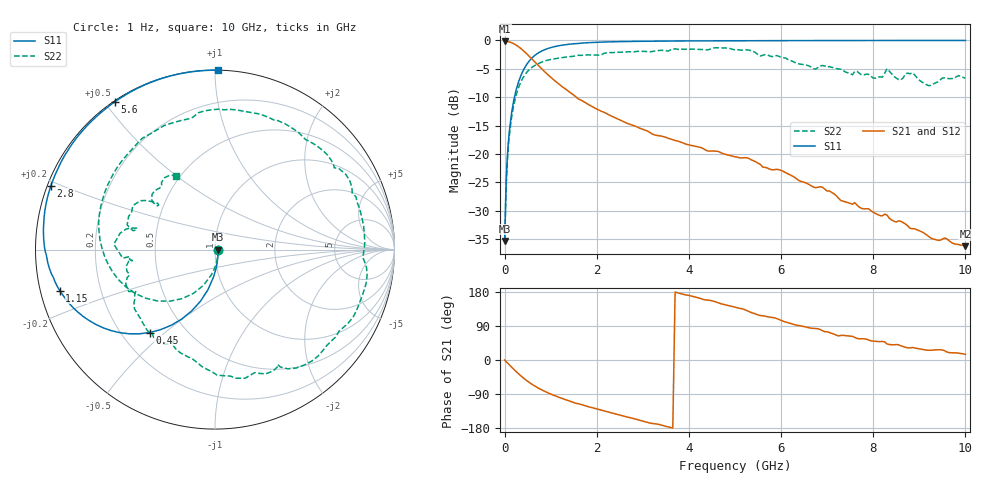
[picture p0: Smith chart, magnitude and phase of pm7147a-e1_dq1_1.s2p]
# GHz S DB R 50
! S-Parameters data
! Freq  dbS11  angS11  dbS21  angS21  dbS12  angS12  dbS22  angS22
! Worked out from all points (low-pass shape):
!   279 points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, 1 Hz to 10 GHz, reference 50 ohm
!   highest |S21| = -0.15 dB at 1.259 kHz (marker M1); lowest = -36.2 dB at 10 GHz (marker M2)
!   |S21| within 3 dB of the highest: start of sweep to 578.2 MHz
!   lowest |S11| = -35.3 dB at 1.585 kHz (marker M3), VSWR 1.03, Z = 51.7 - j0.000223 ohm
!   |S11| at or under -10 dB: start of sweep to 213.7 MHz
!   |S22| runs from -35.3 to -1.3 dB; largest |S21 - S12| = 0
!   S11 on the Smith chart (normalised r, x): 1 Hz: 1.03, -0.00; 450 MHz: 0.31, -0.45; 1.15 GHz: 0.06, -0.13; 2.8 GHz: 0.01, +0.19; 5.6 GHz: 0.00, +0.53; 10 GHz: 0.00, +1.02
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1e-09  -35.30 -0.0  -0.15 -0.0  -0.15 -0.0  -35.30 -0.0
1.2589e-06  -35.30 -0.0  -0.15 -0.0  -0.15 -0.0  -35.30 -0.0
1.5849e-06  -35.30 -0.0  -0.15 -0.0  -0.15 -0.0  -35.30 -0.0
0.03981072  -23.85 -78.0  -0.17 -5.0  -0.17 -5.0  -24.54 -78.8
0.1  -16.21 -93.3  -0.26 -12.5  -0.26 -12.5  -16.95 -98.2
0.25  -8.73 -110.9  -0.81 -30.5  -0.81 -30.5  -9.63 -124.0
0.45  -4.60 -128.3  -2.12 -51.6  -2.12 -51.6  -5.92 -150.9
0.75  -2.11 -148.0  -4.56 -75.4  -4.56 -75.4  -4.00 179.0
1.15  -0.97 -165.2  -7.50 -97.1  -7.50 -97.1  -3.14 149.5
1.7  -0.45 179.5  -10.69 -118.9  -10.69 -118.9  -2.62 117.6
2.8  -0.17 158.7  -14.99 -154.6  -14.99 -154.6  -2.01 65.3
3.35  -0.12 150.6  -16.78 -170.1  -16.78 -170.1  -1.76 42.3
4.2  -0.07 139.5  -18.74 164.2  -18.74 164.2  -1.56 4.8
5.05  -0.06 129.7  -20.53 137.7  -20.53 137.7  -1.61 -35.7
5.6  -0.04 124.0  -22.28 116.7  -22.28 116.7  -2.62 -61.8
6.1  -0.03 119.1  -23.28 100.1  -23.28 100.1  -3.10 -89.0
6.7  -0.02 113.5  -25.79 83.3  -25.79 83.3  -4.96 -114.6
7.3  -0.01 108.3  -28.17 64.8  -28.17 64.8  -5.08 -143.6
8.25  -0.01 100.8  -30.57 47.6  -30.57 47.6  -5.74 -174.7
8.35  -0.01 100.1  -31.30 40.7  -31.30 40.7  -5.42 170.1
9.2  -0.00 94.1  -34.48 25.7  -34.48 25.7  -7.96 141.6
10  -0.00 89.1  -36.21 14.9  -36.21 14.9  -6.68 117.8
